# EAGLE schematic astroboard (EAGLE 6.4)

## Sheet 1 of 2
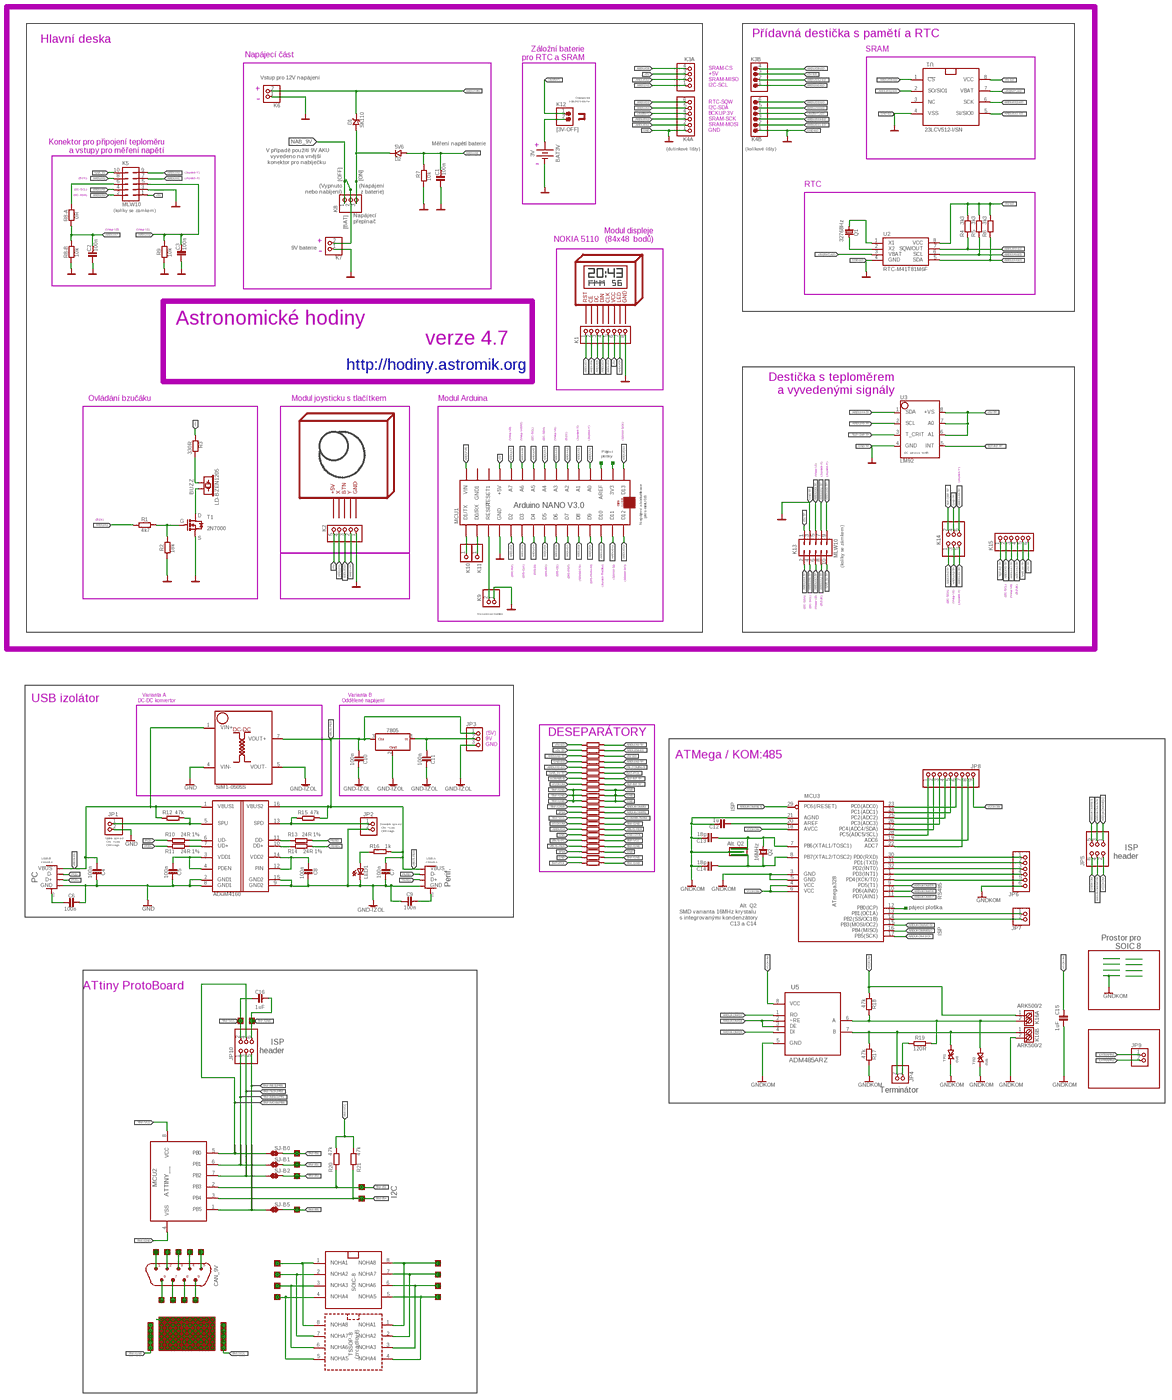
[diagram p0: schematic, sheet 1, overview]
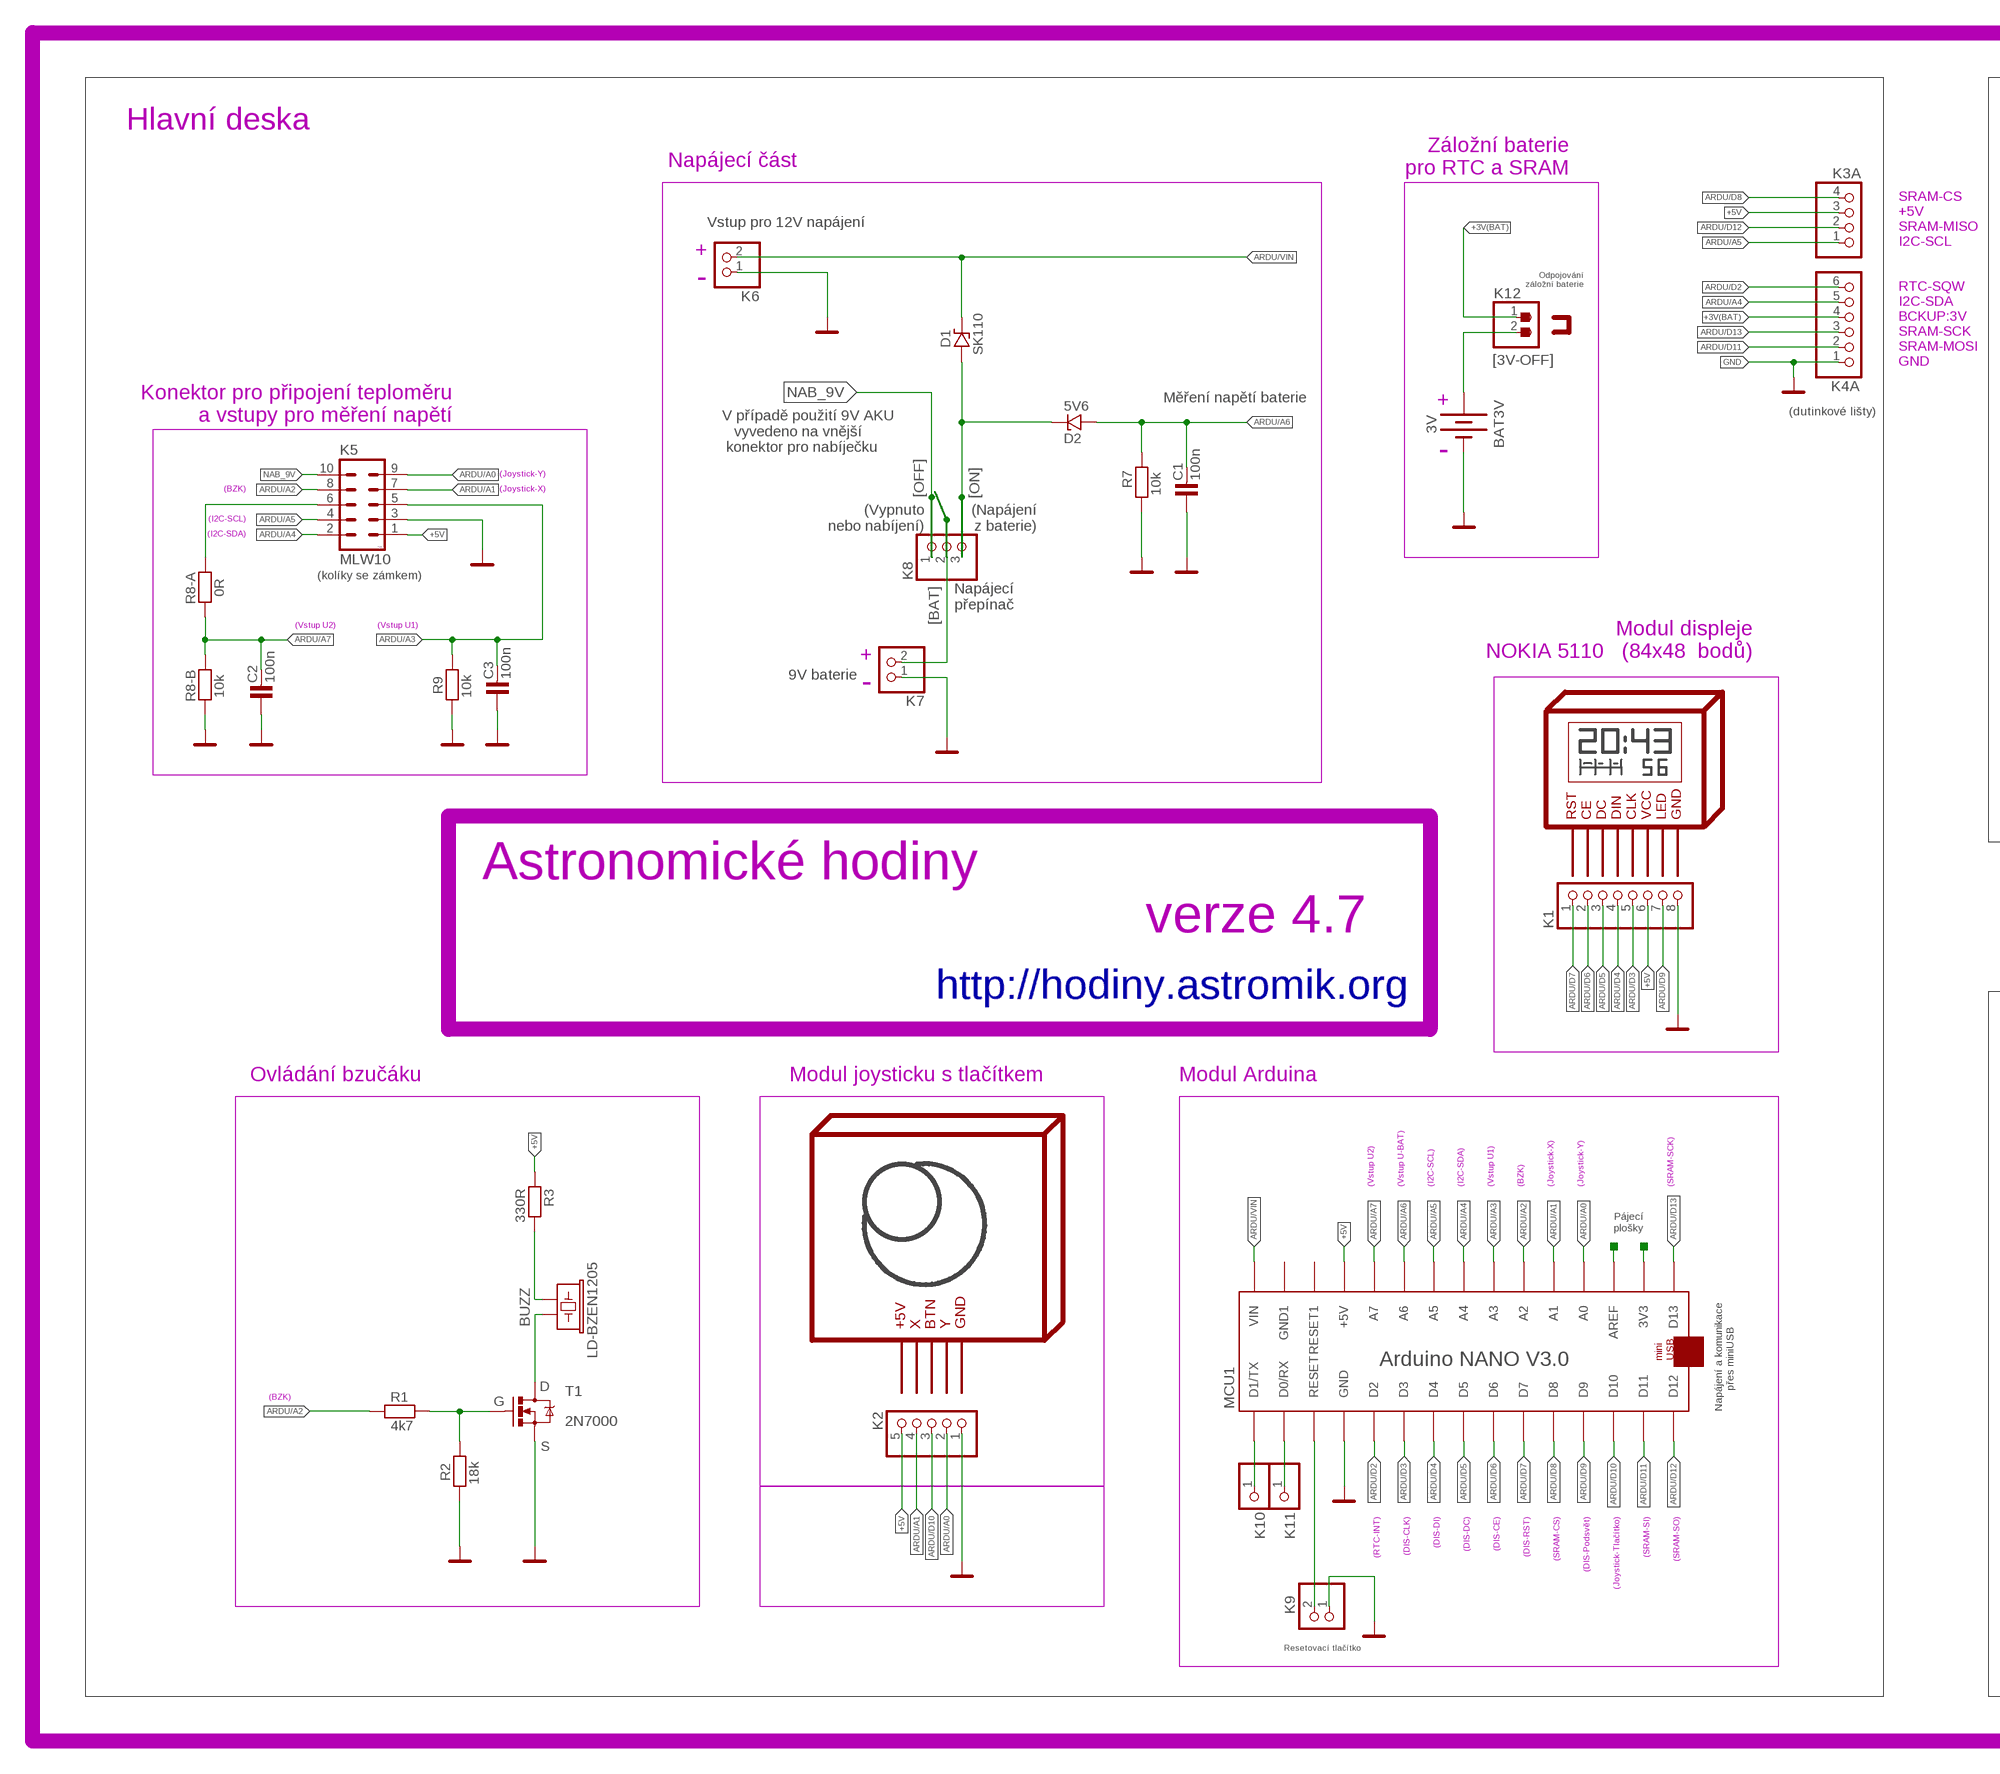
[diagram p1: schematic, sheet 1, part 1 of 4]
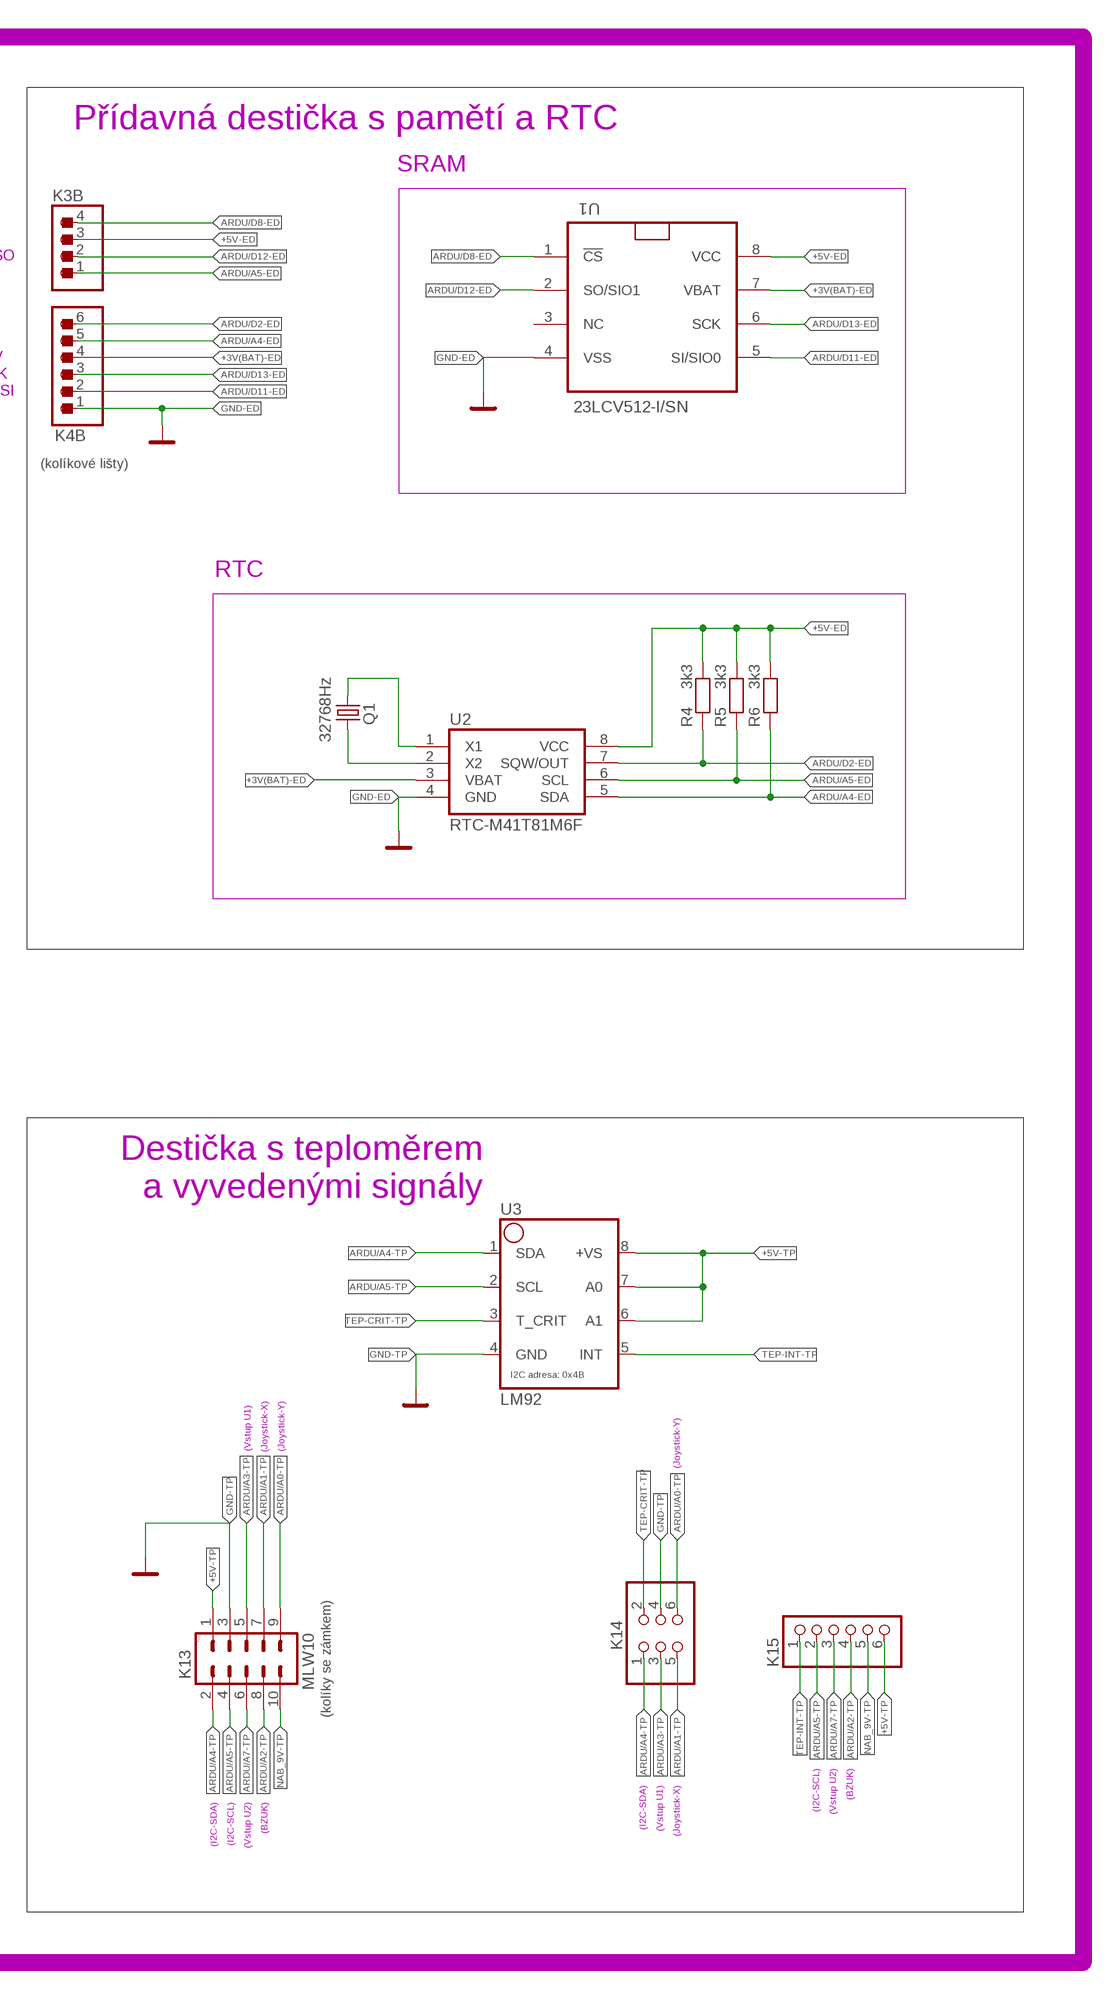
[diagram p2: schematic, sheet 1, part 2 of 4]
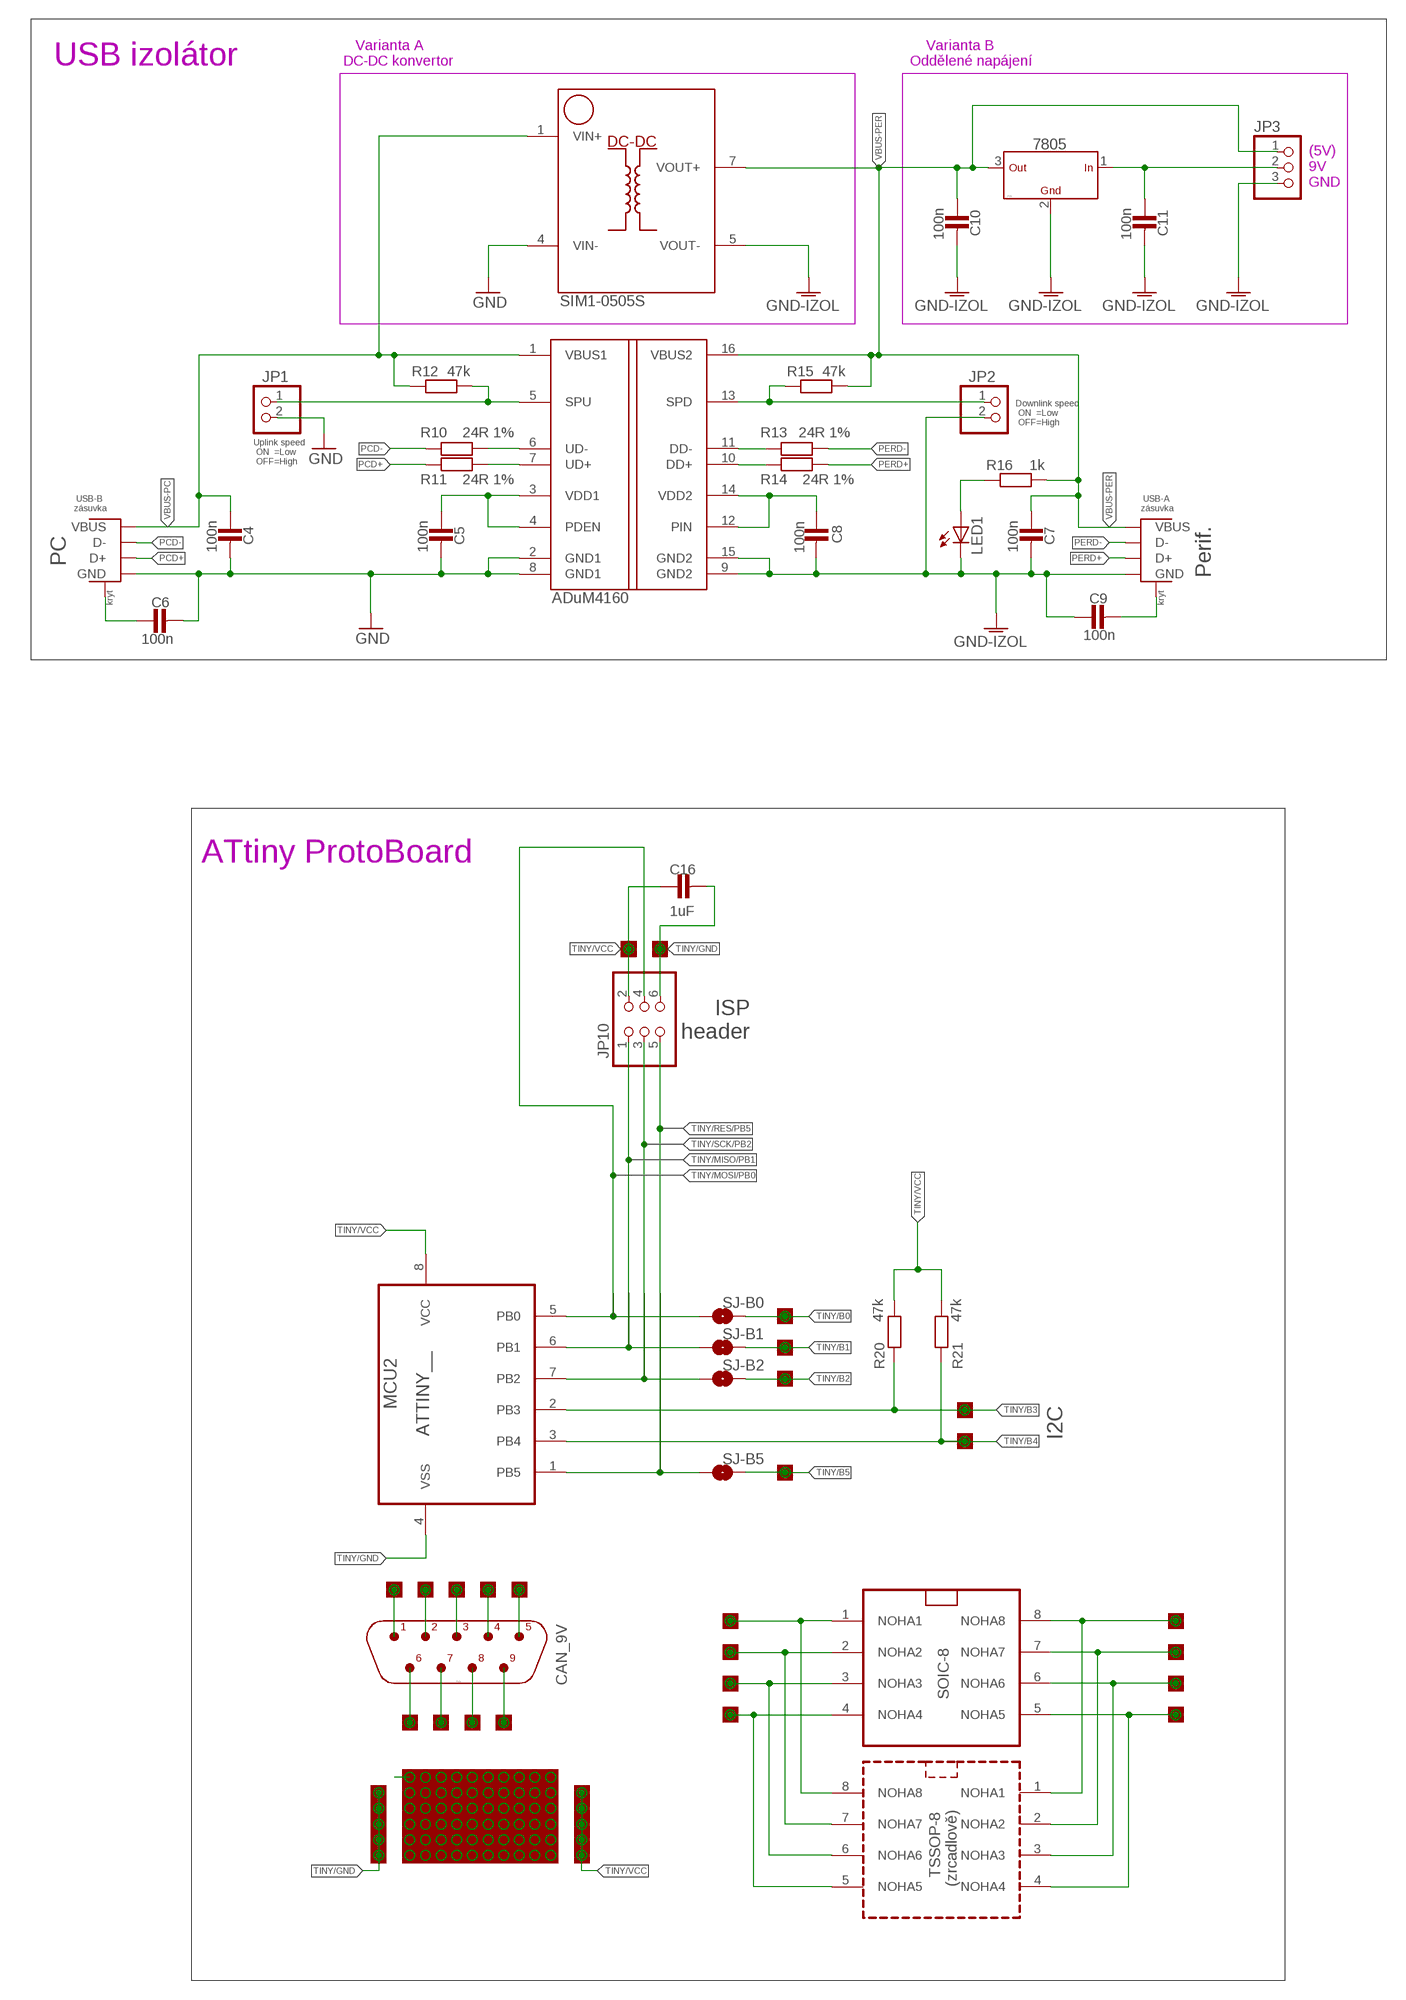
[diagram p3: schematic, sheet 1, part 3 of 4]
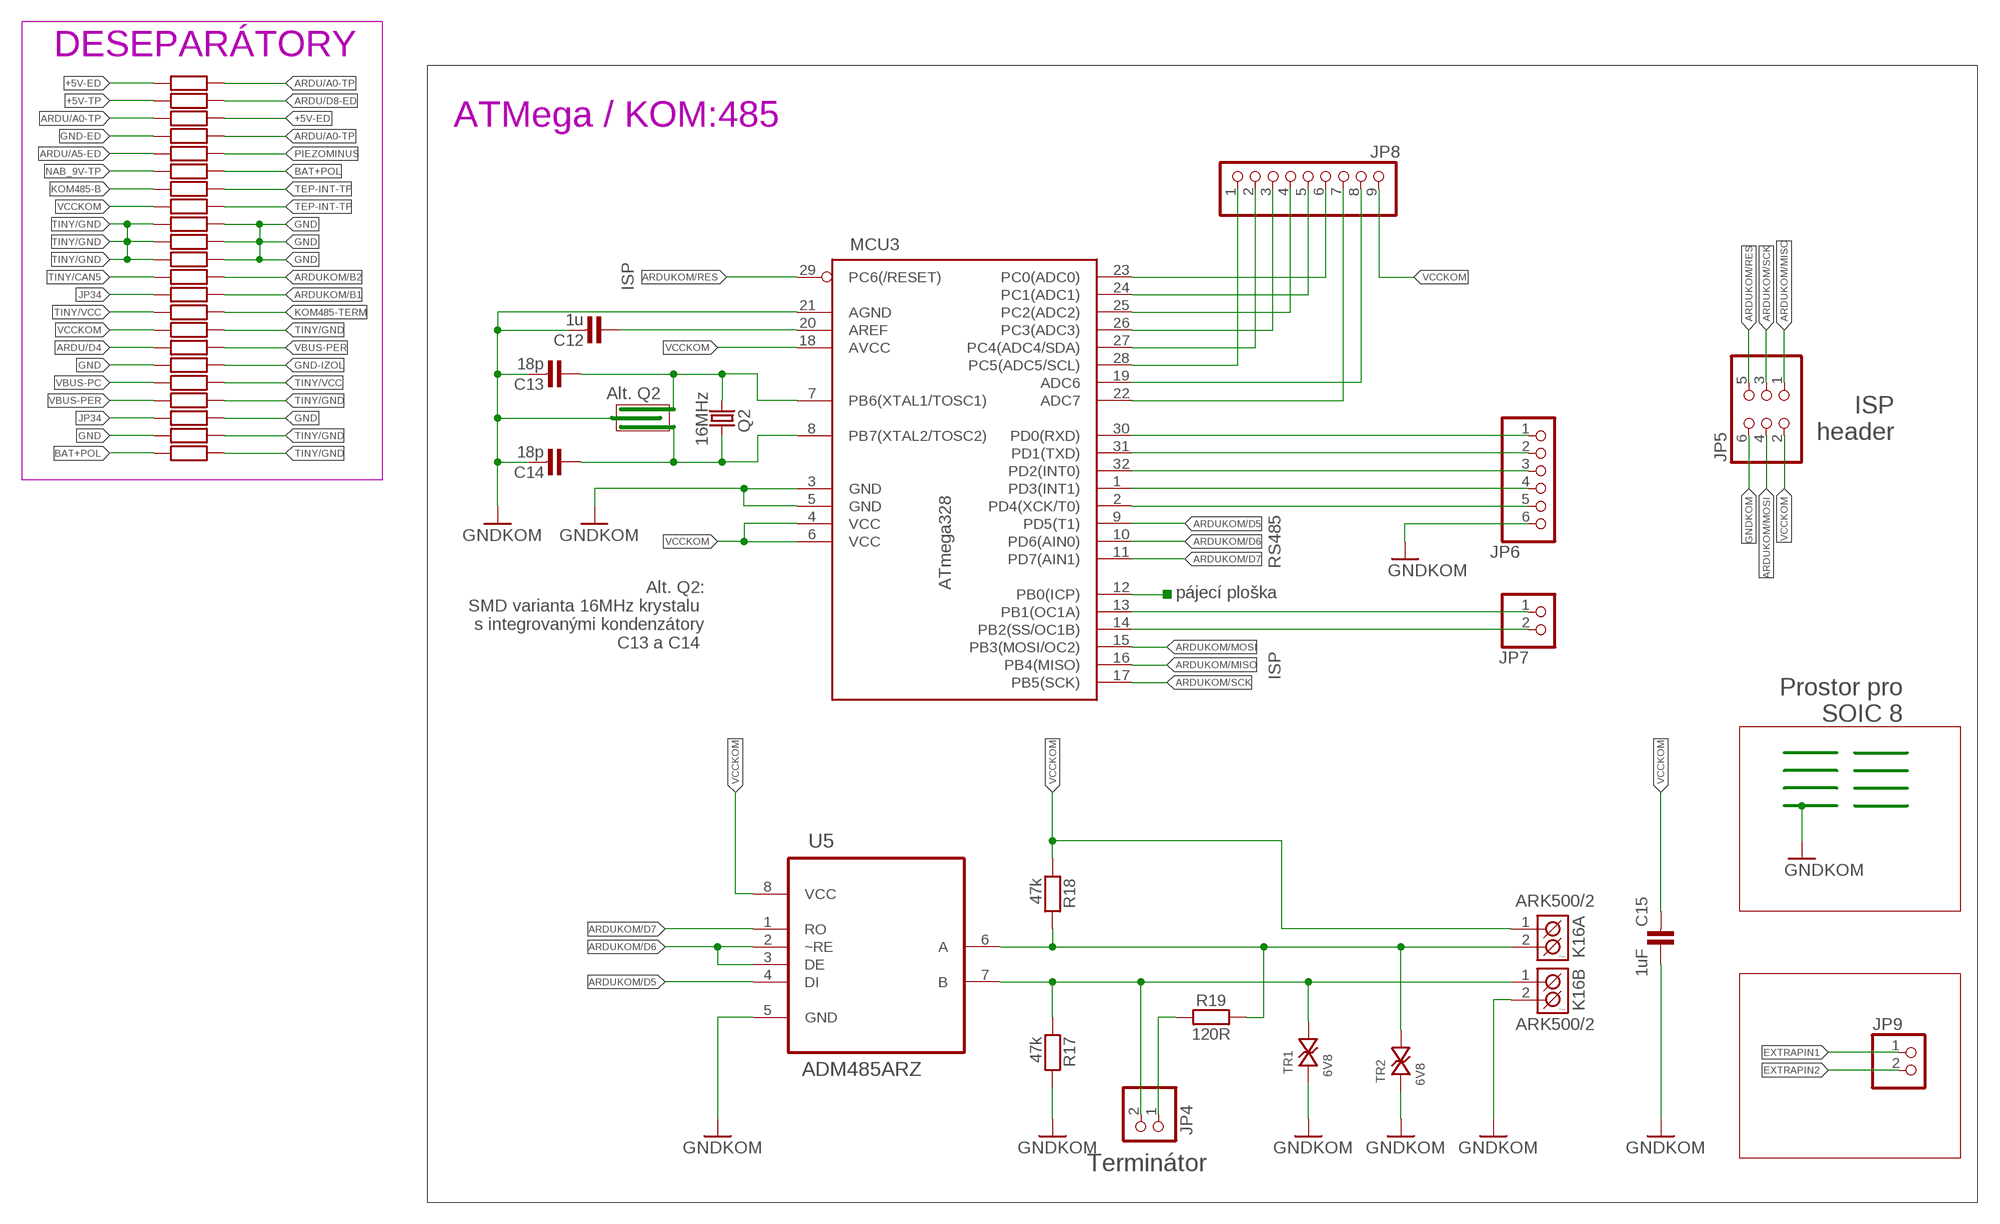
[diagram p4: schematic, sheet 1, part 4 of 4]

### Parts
BAT3V  3V  BATTERY20PTH2  [BATTERY]
BUZZ  LD-BZEN1205  BUZZERNS  [BUZZER-12MM-NS]
C1  100n  C-KERAMIK_SMD_1206  [1206]
C2  100n  C-KERAMIK_SMD_1206  [1206]
C3  100n  C-KERAMIK_SMD_1206  [1206]
C4  100n  C-KERAMIK_SMD_0805  [0805]
C5  100n  C-KERAMIK_SMD_0805  [0805]
C6  100n  C-KERAMIK_SMD_0805  [0805]
C7  100n  C-KERAMIK_SMD_0805  [0805]
C8  100n  C-KERAMIK_SMD_0805  [0805]
C9  100n  C-KERAMIK_SMD_0805  [0805]
C10  100n  C-KERAMIK_SMD_0805  [0805]
C11  100n  C-KERAMIK_SMD_0805  [0805]
C12  1u  C-KERAMIK_SMD_0805  [0805]
C13  18p  C-KERAMIK_SMD_0805  [0805]
C14  18p  C-KERAMIK_SMD_0805  [0805]
C15  1uF  C-KERAMIK_SMD_0805  [0805]
C16  1uF  C-KERAMIK_SMD_0805  [0805]
CAN1  CAN_9V  CAN_9V_/0  [CAN9V]
D1  SK110  1N4007_SM-1  [SM-1]
D2  5V6  D-ZENEROVA_0,5W_BZV55C_SMD  [SOD-80]
DC-DC1  SIM1-0505  [SIM1-0505]
EMPTY1  SOIC-NIC  [SOIC127P600X175-8N]
EMPTY2  TSSOP-NIC  [TSSOP8]
IO1  7805  78_STOJ_STOJ  [TO-220S]
JP1  PINHD-1X2  [1X02]
JP2  PINHD-1X2  [1X02]
JP3  PINHD-1X3  [1X03]
JP4  PINHD-1X2  [1X02]
JP5  PINHD-2X3  [2X03]
JP6  PINHD-1X6  [1X06]
JP7  PINHD-1X2  [1X02]
JP8  PINHD-1X9  [1X09]
JP9  PINHD-1X2  [1X02]
JP10  PINHD-2X3  [2X03]
JP11  PINHD-1X1  [1X01]
JP12  PINHD-1X1  [1X01]
JP13  PINHD-1X1  [1X01]
JP14  PINHD-1X1  [1X01]
JP15  PINHD-1X1  [1X01]
JP16  PINHD-1X1  [1X01]
JP17  PINHD-1X1  [1X01]
JP18  PINHD-1X1  [1X01]
JP19  PINHD-1X1  [1X01]
JP20  PINHD-1X1  [1X01]
JP21  PINHD-1X1  [1X01]
JP22  PINHD-1X1  [1X01]
JP23  PINHD-1X1  [1X01]
JP24  PINHD-1X1  [1X01]
JP25  PINHD-1X1  [1X01]
JP26  PINHD-1X1  [1X01]
JP27  PINHD-1X1  [1X01]
JP28  PINHD-1X1  [1X01]
JP29  PINHD-1X1  [1X01]
JP30  PINHD-1X1  [1X01]
JP31  PINHD-1X1  [1X01]
JP32  PINHD-1X1  [1X01]
JP33  PINHD-1X1  [1X01]
JP34  PINHD-1X1  [1X01]
JP35  PINHD-1X1  [1X01]
JP36  PINHD-1X1  [1X01]
JP37  PINHD-1X1  [1X01]
JP38  PINHD-1X1  [1X01]
JP39  PINHD-1X1  [1X01]
JP40  PINHD-1X1  [1X01]
JP41  PINHD-1X1  [1X01]
JP42  PINHD-1X1  [1X01]
JP43  PINHD-1X1  [1X01]
JP44  PINHD-1X1  [1X01]
JP45  PINHD-1X1  [1X01]
JP46  PINHD-1X1  [1X01]
JP47  PINHD-1X1  [1X01]
JP48  PINHD-1X1  [1X01]
JP49  PINHD-1X1  [1X01]
JP50  PINHD-1X1  [1X01]
JP51  PINHD-1X1  [1X01]
JP52  PINHD-1X1  [1X01]
JP53  PINHD-1X1  [1X01]
JP54  PINHD-1X1  [1X01]
JP55  PINHD-1X1  [1X01]
JP56  PINHD-1X1  [1X01]
JP57  PINHD-1X1  [1X01]
JP58  PINHD-1X1  [1X01]
JP59  PINHD-1X1  [1X01]
JP60  PINHD-1X1  [1X01]
JP61  PINHD-1X1  [1X01]
JP62  PINHD-1X1  [1X01]
JP63  PINHD-1X1  [1X01]
JP64  PINHD-1X1  [1X01]
JP65  PINHD-1X1  [1X01]
JP66  PINHD-1X1  [1X01]
JP67  PINHD-1X1  [1X01]
JP68  PINHD-1X1  [1X01]
JP69  PINHD-1X1  [1X01]
JP70  PINHD-1X1  [1X01]
JP71  PINHD-1X1  [1X01]
JP72  PINHD-1X1  [1X01]
JP73  PINHD-1X1  [1X01]
JP74  PINHD-1X1  [1X01]
JP75  PINHD-1X1  [1X01]
JP76  PINHD-1X1  [1X01]
JP77  PINHD-1X1  [1X01]
JP78  PINHD-1X1  [1X01]
JP79  PINHD-1X1  [1X01]
JP80  PINHD-1X1  [1X01]
JP81  PINHD-1X1  [1X01]
JP82  PINHD-1X1  [1X01]
JP83  PINHD-1X1  [1X01]
JP84  PINHD-1X1  [1X01]
JP85  PINHD-1X1  [1X01]
JP86  PINHD-1X1  [1X01]
JP87  PINHD-1X1  [1X01]
JP88  PINHD-1X1  [1X01]
JP89  PINHD-1X1  [1X01]
JP90  PINHD-1X1  [1X01]
JP91  PINHD-1X1  [1X01]
JP92  PINHD-1X1  [1X01]
JP93  PINHD-1X1  [1X01]
JP94  PINHD-1X1  [1X01]
JP95  PINHD-1X1  [1X01]
JP97  PINHD-1X1  [1X01]
JP98  PINHD-1X1  [1X01]
JP99  PINHD-1X1  [1X01]
JP100  PINHD-1X1  [1X01]
JP101  PINHD-1X1  [1X01]
JP103  PINHD-1X1  [1X01]
JP104  PINHD-1X1  [1X01]
JP105  PINHD-1X1  [1X01]
JP106  PINHD-1X1  [1X01]
JP108  PINHD-1X1  [1X01]
K1  PINHD-1X8  [1X08]
K2  PINHD-1X5  [1X05]
K3A  PINHD-1X4  [1X04]
K3B  PINHD-1X4  [1X04]
K4A  PINHD-1X6  [1X06]
K4B  PINHD-1X6  [1X06]
K5  MLW10  [MLW10G]
K6  PINHD-1X2  [1X02]
K7  HEADER-1X2  [1X02_OVAL]
K8  PINHD-1X3  [1X03]
K9  PINHD-1X2  [1X02]
K10  PINHD-1X1  [1X01]
K11  PINHD-1X1  [1X01]
K12  PINHD-1X2  [1X02]
K13  MLW10  [MLW10G]
K14  PINHD-2X3  [2X03]
K15  PINHD-1X6  [1X06]
K16A  ARK500/2  [ARK500/2]
K16B  ARK500/2  [ARK500/2]
LED1  LEDCHIP-LED0805  [CHIP-LED0805]
MCU1  ARDUINONANO  [PDIP-32]
MCU2  ATTINY__  ATTINY13  [SOIC127P600X175-8N]
MCU3  ATmega328  MEGA8-AI  [TQFP32-08]
Q1  32768Hz  CRYSTALTC26V  [TC26V]
Q2  16MHz  CRYSTALHC49U-V  [HC49U-V]
R1  4k7  R_SMD_1206  [1206]
R2  18k  R_SMD_1206  [1206]
R3  330R  R_SMD_1206  [1206]
R4  3k3  R_SMD_1206  [1206]
R5  3k3  R_SMD_1206  [1206]
R6  3k3  R_SMD_1206  [1206]
R7  10k  R_SMD_1206  [1206]
R8  1k  R_SMD_1206  [1206]
R8-A  0R  R_SMD_1206  [1206]
R8-B  10k  R_SMD_1206  [1206]
R9  10k  R_SMD_1206  [1206]
R10  24R 1%  R_SMD_0805  [0805]
R11  24R 1%  R_SMD_0805  [0805]
R12  47k  R_SMD_0805  [0805]
R13  24R 1%  R_SMD_0805  [0805]
R14  24R 1%  R_SMD_0805  [0805]
R15  47k  R_SMD_0805  [0805]
R16  1k  R_SMD_0805  [0805]
R17  47k  R_SMD_0805  [0805]
R18  47k  R_SMD_0805  [0805]
R19  120R  R_SMD_0805  [0805]
R20  47k  R_SMD_0805  [0805]
R21  47k  R_SMD_0805  [0805]
R22  1k  R_SMD_1206  [1206]
R23  1k  R_SMD_1206  [1206]
R24  1k  R_SMD_1206  [1206]
R25  1k  R_SMD_1206  [1206]
R26  1k  R_SMD_1206  [1206]
R27  1k  R_SMD_1206  [1206]
R28  1k  R_SMD_1206  [1206]
R29  1k  R_SMD_1206  [1206]
R30  1k  R_SMD_1206  [1206]
R31  1k  R_SMD_1206  [1206]
R32  1k  R_SMD_1206  [1206]
R33  1k  R_SMD_1206  [1206]
R34  1k  R_SMD_1206  [1206]
R35  1k  R_SMD_1206  [1206]
R36  1k  R_SMD_1206  [1206]
R37  1k  R_SMD_1206  [1206]
R38  1k  R_SMD_1206  [1206]
R39  1k  R_SMD_1206  [1206]
R40  1k  R_SMD_1206  [1206]
R41  1k  R_SMD_1206  [1206]
R42  1k  R_SMD_1206  [1206]
SJ-B0  SOLDERJUMPERNC  [SJ-NC]
SJ-B1  SOLDERJUMPERNC  [SJ-NC]
SJ-B2  SOLDERJUMPERNC  [SJ-NC]
SJ-B5  SOLDERJUMPERNC  [SJ-NC]
T1  2N7000  MOSFET-NCHANNELPTH  [TO-92]
TR1  6V8  SMAJ30CA-TR__DO214AC+MINIMELF  [DO214AC+MINIMELF_BIDIR]
TR2  6V8  SMAJ30CA-TR__DO214AC+MINIMELF  [DO214AC+MINIMELF_BIDIR]
U1  23LCV512-I/SN  [SOIC127P600X175-8N]
U2  RTC-M41T81M6F  IC_RTC_DS1307  [SO-8]
U3  LM92  [SO08]
U4  ADuM4160  ADUM4160  [SO16W]
U5  ADM485ARZ  [SOIC127P600X175-8N]
X1  USB B  USBPTH  [USB-B-PTH]
X2  USB A  USBA-H  [USB-A-H]

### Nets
+3V(BAT): K4A.4 K12.1
+3V(BAT)-ED: K4B.4 U1.7(VBAT) U2.3(VBAT)
+5V: K1.6 K2.5 K3A.3 K5.1 MCU1.+5V R3.1
+5V-ED: K3B.3 R4.2 R5.2 R6.2 R8.1 R33.2 U1.8(VCC) U2.8(VCC)
+5V-TP: K13.1 K15.6 R25.2 U3.6(A1) U3.7(A0) U3.8(+VS)
ARDU/3V3: MCU1.3V3
ARDU/A0: K2.2 K5.9 MCU1.A0
ARDU/A0-TP: K13.9 K14.6 R8.2 R22.1 R33.1
ARDU/A1: K2.4 K5.7 MCU1.A1
ARDU/A1-TP: K13.7 K14.5
ARDU/A2: K5.8 MCU1.A2 R1.1
ARDU/A2-TP: K13.8 K15.4
ARDU/A3: C3.2 K5.5 MCU1.A3 R9.2
ARDU/A3-TP: K13.5 K14.3
ARDU/A4: K4A.5 K5.2 MCU1.A4
ARDU/A4-ED: K4B.5 R6.1 U2.5(SDA)
ARDU/A4-TP: K13.2 K14.1 U3.1(SDA)
ARDU/A5: K3A.1 K5.4 MCU1.A5
ARDU/A5-ED: K3B.1 R5.1 R23.2 U2.6(SCL)
ARDU/A5-TP: K13.4 K15.2 U3.2(SCL)
ARDU/A6: C1.2 D2.A MCU1.A6 R7.2
ARDU/A7: C2.2 MCU1.A7 R8-A.1 R8-B.2
ARDU/A7-TP: K13.6 K15.3
ARDU/AREF: MCU1.AREF
ARDU/D0: K11.1 MCU1.D0/RX
ARDU/D1: K10.1 MCU1.D1/TX
ARDU/D2: K4A.6 MCU1.D2
ARDU/D2-ED: K4B.6 R4.1 U2.7(SQW/OUT)
ARDU/D3: K1.5 MCU1.D3
ARDU/D4: K1.4 MCU1.D4 R36.2
ARDU/D5: K1.3 MCU1.D5
ARDU/D6: K1.2 MCU1.D6
ARDU/D7: K1.1 MCU1.D7
ARDU/D8: K3A.4 MCU1.D8
ARDU/D8-ED: K3B.4 R25.1 U1.1(!CS)
ARDU/D9: K1.7 MCU1.D9
ARDU/D10: K2.3 MCU1.D10
ARDU/D11: K4A.2 MCU1.D11
ARDU/D11-ED: K4B.2 U1.5(SI/SIO0)
ARDU/D12: K3A.2 MCU1.D12
ARDU/D12-ED: K3B.2 U1.2(SO/SIO1)
ARDU/D13: K4A.3 MCU1.D13
ARDU/D13-ED: K4B.3 U1.6(SCK)
ARDU/RESET: K9.2 MCU1.RESET
ARDU/VIN: D1.K K6.2 MCU1.VIN
ARDUKOM/B0: MCU3.12(PB0(ICP))
ARDUKOM/B1: JP7.1 MCU3.13(PB1(OC1A)) R32.1
ARDUKOM/B2: JP7.2 MCU3.14(PB2(SS/OC1B)) R30.1
ARDUKOM/C0: JP8.6 MCU3.23(PC0(ADC0))
ARDUKOM/C1: JP8.5 MCU3.24(PC1(ADC1))
ARDUKOM/C2: JP8.4 MCU3.25(PC2(ADC2))
ARDUKOM/C3: JP8.3 MCU3.26(PC3(ADC3))
ARDUKOM/C4: JP8.2 MCU3.27(PC4(ADC4/SDA))
ARDUKOM/C5: JP8.1 MCU3.28(PC5(ADC5/SCL))
ARDUKOM/C6: JP8.8 MCU3.19(ADC6)
ARDUKOM/C7: JP8.7 MCU3.22(ADC7)
ARDUKOM/D0: JP6.1 MCU3.30(PD0(RXD))
ARDUKOM/D1: JP6.2 MCU3.31(PD1(TXD))
ARDUKOM/D2: JP6.3 MCU3.32(PD2(INT0))
ARDUKOM/D3: JP6.4 MCU3.1(PD3(INT1))
ARDUKOM/D4: JP6.5 MCU3.2(PD4(XCK/T0))
ARDUKOM/D5: MCU3.9(PD5(T1)) U5.4(DI)
ARDUKOM/D6: MCU3.10(PD6(AIN0)) U5.2(~RE) U5.3(DE)
ARDUKOM/D7: MCU3.11(PD7(AIN1)) U5.1(RO)
ARDUKOM/MISO: JP5.1 MCU3.16(PB4(MISO))
ARDUKOM/MOSI: JP5.4 MCU3.15(PB3(MOSI/OC2))
ARDUKOM/RES: JP5.5 MCU3.29(PC6(/RESET))
ARDUKOM/SCK: JP5.3 MCU3.17(PB5(SCK))
BAT+POL: BAT3V.+ K12.2 R24.1 R42.2
BZUK/GATE: R1.2 R2.2 T1.3(G)
EXTRAPIN1: JP9.1
EXTRAPIN2: JP9.2
GND: BAT3V.- C1.1 C2.1 C3.1 K1.8 K2.1 K4A.1 K5.3 K6.1 K7.1 K9.1 MCU1.GND R2.1 R7.1 R8-B.1 R9.1 R27.1 R28.1 R29.1 R37.2 R40.1 R41.2 T1.1(S)
GND-ED: K4B.1 R22.2 U1.4(VSS) U2.4(GND) ; supply symbol labelled GND
GND-IZOL: C7.2 C8.2 C9.1 C10.2 C11.2 DC-DC1.5(VOUT-) IO1.2(GND) JP2.2 JP3.3 LED1.C R37.1 U4.9(GND2) U4.15(GND2) X2.GND
GND-PC: C4.2 C5.2 C6.2 DC-DC1.4(VIN-) JP1.2 U4.2(GND1) U4.8(GND1) X1.GND ; supply symbol labelled GND
GND-TP: K13.3 K14.4 U3.4(GND) ; supply symbol labelled GND
GNDKOM: C12.2 C13.2 C14.2 C15.1 JP5.6 JP6.6 K16B.2(K2) MCU3.3(GND) MCU3.5(GND) MCU3.21(AGND) R17.2 TR1.P$1 TR2.P$1 U5.5(GND)
JP34: JP34.1 R32.2 R40.2
KOM485-A: K16A.2(K2) R18.2 R19.2 TR2.P$2 U5.6(A)
KOM485-B: JP4.2 K16B.1(K1) R17.1 R26.2 TR1.P$2 U5.7(B)
KOM485-TERM: JP4.1 R19.1 R34.1
N$1: K5.6 R8-A.2
N$2: C6.1 X1.P$2(SHIELD)
N$3: R11.2 U4.7(UD+)
N$4: R10.2 U4.6(UD-)
N$5: C9.2 X2.SHIELD@1(SHIELD)
N$9: JP1.1 R12.1 U4.5(SPU)
N$10: JP2.1 R15.1 U4.13(SPD)
N$14: R14.1 U4.10(DD+)
N$15: C11.1 IO1.1(IN) JP3.2
N$16: R13.1 U4.11(DD-)
N$18: LED1.A R16.1
N$21: C13.1 MCU3.7(PB6(XTAL1/TOSC1)) Q2.2
N$22: C14.1 MCU3.8(PB7(XTAL2/TOSC2)) Q2.1
N$28: C12.1 MCU3.20(AREF)
NAB_9V: K5.10 K8.1
NAB_9V-TP: K13.10 K15.5 R24.2
NAPETI_9V: D1.A D2.K K8.3
OSC1-ED: Q1.2 U2.1(X1)
OSC2-ED: Q1.1 U2.2(X2)
PCD+: R11.1 X1.D+
PCD-: R10.1 X1.D-
PERD+: R14.2 X2.D+
PERD-: R13.2 X2.D-
PIEZOMINUS: BUZZ.- R23.1 T1.2(D)
PIEZOPLUS: BUZZ.+ R3.2
PLUS_9V: K7.2 K8.2
TEP-CRIT-TP: K14.2 U3.3(T_CRIT)
TEP-INT-TP: K15.1 R26.1 R31.1 U3.5(INT)
TINY/B0: JP27.1 SJ-B0.2
TINY/B1: JP28.1 SJ-B1.2
TINY/B2: JP29.1 SJ-B2.2
TINY/B3: JP31.1 MCU2.2(PB3) R20.1
TINY/B4: JP32.1 MCU2.3(PB4) R21.1
TINY/B5: JP30.1 SJ-B5.2
TINY/CAN1: CAN1.1 JP18.1
TINY/CAN2: CAN1.2 JP19.1
TINY/CAN3: CAN1.3 JP20.1
TINY/CAN4: CAN1.4 JP21.1
TINY/CAN5: CAN1.5 JP22.1 R30.2
TINY/CAN6: CAN1.6 JP23.1
TINY/CAN7: CAN1.7 JP24.1
TINY/CAN8: CAN1.8 JP25.1
TINY/CAN9: CAN1.9 JP26.1
TINY/GND: C16.2 JP10.6 JP93.1 JP94.1 JP97.1 JP98.1 JP99.1 JP100.1 MCU2.4(VSS) R27.2 R28.2 R29.2 R35.1 R39.1 R41.1 R42.1
TINY/MISO/PB1: JP10.1 MCU2.6(PB1) SJ-B1.1
TINY/MOSI/PB0: JP10.4 MCU2.5(PB0) SJ-B0.1
TINY/RES/PB5: JP10.5 MCU2.1(PB5) SJ-B5.1
TINY/SCK/PB2: JP10.3 MCU2.7(PB2) SJ-B2.1
TINY/SOIC1: EMPTY1.1(NOHA1) EMPTY2.8(NOHA8) JP14.1
TINY/SOIC2: EMPTY1.2(NOHA2) EMPTY2.7(NOHA7) JP15.1
TINY/SOIC3: EMPTY1.3(NOHA3) EMPTY2.6(NOHA6) JP16.1
TINY/SOIC4: EMPTY1.4(NOHA4) EMPTY2.5(NOHA5) JP17.1
TINY/SOIC5: EMPTY1.5(NOHA5) EMPTY2.4(NOHA4) JP13.1
TINY/SOIC6: EMPTY1.6(NOHA6) EMPTY2.3(NOHA3) JP12.1
TINY/SOIC7: EMPTY1.7(NOHA7) EMPTY2.2(NOHA2) JP11.1
TINY/SOIC8: EMPTY1.8(NOHA8) EMPTY2.1(NOHA1) JP108.1
TINY/VCC: C16.1 JP10.2 JP95.1 JP101.1 JP103.1 JP104.1 JP105.1 JP106.1 MCU2.8(VCC) R20.2 R21.2 R34.2 R38.1
VBUS-PC: C4.1 DC-DC1.1(VIN+) R12.2 R38.2 U4.1(VBUS1) X1.VBUS
VBUS-PER: C7.1 C10.1 DC-DC1.7(VOUT+) IO1.3(OUT) JP3.1 R15.2 R16.2 R36.1 R39.2 U4.16(VBUS2) X2.VBUS
VCCKOM: C15.2 JP5.2 JP8.9 K16A.1(K1) MCU3.4(VCC) MCU3.6(VCC) MCU3.18(AVCC) R18.1 R31.2 R35.2 U5.8(VCC)
VDD1: C5.1 U4.3(VDD1) U4.4(PDEN)
VDD2: C8.1 U4.12(PIN) U4.14(VDD2)
Unconnected: JP33.1 JP35.1 JP36.1 JP37.1 JP38.1 JP39.1 JP40.1 JP41.1 JP42.1 JP43.1 JP44.1 JP45.1 JP46.1 JP47.1 JP48.1 JP49.1 JP50.1 JP51.1 JP52.1 JP53.1 JP54.1 JP55.1 JP56.1 JP57.1 JP58.1 JP59.1 JP60.1 JP61.1 JP62.1 JP63.1 JP64.1 JP65.1 JP66.1 JP67.1 JP68.1 JP69.1 JP70.1 JP71.1 JP72.1 JP73.1 JP74.1 JP75.1 JP76.1 JP77.1 JP78.1 JP79.1 JP80.1 JP81.1 JP82.1 JP83.1 JP84.1 JP85.1 JP86.1 JP87.1 JP88.1 JP89.1 JP90.1 JP91.1 JP92.1 MCU1.GND1 MCU1.RESET1 U1.3(NC)

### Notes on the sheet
- Přídavná destička s pamětí a RTC
- Hlavní deska
- Záložní baterie
   pro RTC a SRAM
- SRAM
- Napájecí část
- SRAM-CS
- +5V
- Vstup pro 12V napájení | SRAM-MISO
- + | I2C-SCL
- -
- Odpojování
   záložní baterie
- RTC-SQW
- I2C-SDA
- BCKUP:3V
- SRAM-SCK
- [3V-OFF] | SRAM-MOSI
- GND
- Konektor pro připojení teploměru
  a vstupy pro měření napětí
- Měření napětí baterie | +
- (dutinkové lišty) | (kolíkové lišty)
- -
- V případě použití 9V AKU
     vyvedeno na vnější
   konektor pro nabíječku
- [ON]
- (Joystick-Y)
- (BZK) | (Joystick-X)
- [OFF] | RTC
- (Vypnuto
   nebo nabíjení)
- (Napájení
  z baterie)
- (I2C-SCL)
- (I2C-SDA)
- (kolíky se zámkem)
- Napájecí
  přepínač
- Modul displeje
  NOKIA 5110   (84x48  bodů)
- [BAT]
- (Vstup U2) | (Vstup U1)
- +
- 9V baterie | -
- RST | CE | DC | DIN | CLK | VCC | LED | GND
- Astronomické hodiny | verze 4.7
- http://hodiny.astromik.org
- Destička s teploměrem
  a vyvedenými signály
- Ovládání bzučáku | Modul joysticku s tlačítkem | Modul Arduina
- (Vstup U2) | (Vstup U-BAT) | (I2C-SCL) | (I2C-SDA) | (Vstup U1) | (BZK) | (Joystick-X) | (Joystick-Y) | (SRAM-SCK)
- I2C adresa: 0x4B
- Pájecí
  plošky
- (Joystick-X) | (Joystick-Y)
- (Vstup U1)
- (Joystick-Y)
- +5V | X | BTN | Y | GND
- Arduino NANO V3.0
- MCU1
- D
- G
- (BZK)
- Napájení a komunikace
         přes miniUSB
- S
- (RTC-INT) | (DIS-CLK) | (DIS-DI) | (DIS-DC) | (DIS-CE) | (DIS-RST) | (SRAM-CS) | (DIS-Podsvět) | (Joystick-Tlačítko) | (SRAM-SI) | (SRAM-SO)
- (kolíky se zámkem)
- (I2C-SCL) | (Vstup U2) | (BZUK)
- (I2C-SDA) | (Vstup U1) | (Joystick-X)
- (I2C-SDA) | (I2C-SCL) | (Vstup U2) | (BZUK)
- Resetovací tlačítko
- USB izolátor
- Varianta A
  DC-DC konvertor
- Varianta B
  Oddělené napájení
- DESEPARÁTORY
- (5V)
- 9V
- GND
- ATMega / KOM:485
- ISP
- Downlink speed
   ON  =Low
   OFF=High
- Alt. Q2
- ISP
  header
- Uplink speed
   ON  =Low
   OFF=High
- USB-B
  zásuvka
- USB-A
  zásuvka
- PC | RS485
- Perif.
- kryt | kryt
- Alt. Q2:
    SMD varianta 16MHz krystalu 
    s integrovanými kondenzátory
    C13 a C14
- pájecí ploška
- ISP
- Prostor pro
     SOIC 8
- ATtiny ProtoBoard
- ISP
  header
- Terminátor
- I2C
- SOIC-8
- TSSOP-8
  (zrcadlově)

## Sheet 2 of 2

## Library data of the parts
BAT3V = SparkFun:BATTERY: Battery Holders
BUZZ = SparkFun:BUZZER: Buzzer 12mm
C1-C16 = #PaJa_30:C-KERAMIK: Kondenzator - keramicky
CAN1 = #PaJa_konektory:CAN_9V: Konektory CANNON - vidlice - 9pinu
D1 = #PaJa_30:1N4007: Usmernovaci dioda - 1A, 1000V
D2 = #PaJa_30:D-ZENEROVA: Zenerova dioda
DC-DC1 = sim1-0505:SIM1-0505: DC-DC converter 5V/200mA
EMPTY1 = soic-nic:SOIC-NIC: SOIC-NIC; PACKAGE: SOIC-8
EMPTY2 = tssop-nic:TSSOP-NIC: TSSOP-NIC; PACKAGE: TSSOP-8
IO1 = #PaJa_30:78??: Stabilizátor - 1A a 1,5A ?? - napeti => 05, 06, 08, 09, 12, 15, 18, 20, 24 => 1,5A ?? - napeti => 10, 12, 15, 18 => 1A S ?? - napeti => 05, 09, 10, 12, 15, 18, 24 => 2A T ?? - napeti => 05 => 3A
JP1 JP2 JP4 JP7 JP9 K6 K9 = pinhead:PINHD-1X2: PIN HEADER
JP3 K8 = pinhead:PINHD-1X3: PIN HEADER
JP5 JP10 K14 = pinhead:PINHD-2X3: PIN HEADER
JP6 K4A K15 = pinhead:PINHD-1X6: PIN HEADER
JP8 = pinhead:PINHD-1X9: PIN HEADER
JP11-JP95 JP97-JP101 JP103-JP106 JP108 = jedenpin:PINHD-1X1: PIN HEADER
K1 = pinhead:PINHD-1X8: PIN HEADER
K2 = pinhead:PINHD-1X5: PIN HEADER
K3A = pinhead:PINHD-1X4: PIN HEADER
K3B = pinhead-rev:PINHD-1X4: PIN HEADER
K4B = pinhead-rev:PINHD-1X6: PIN HEADER
K5 K13 = #PaJa_konektory:MLW10: Konektory MLW - vidlice - 10x
K7 = nonolith:HEADER-1X2: PIN HEADER
K10 K11 = pinhead:PINHD-1X1: PIN HEADER
K12 = pinhead-rev:PINHD-1X2: PIN HEADER
K16A K16B = #PaJa_konektory:ARK500/2: Svorkovnice - roztec 5mm - dvojita
LED1 = adafruit:LED: LED
MCU1 = jet-lib:ARDUINONANO
MCU2 = ATTiny13:ATTINY13: ATTINY13; PACKAGE: SOIC-8
MCU3 = avr:MEGA8: MICROCONTROLLER 8 Kbytes FLASH 1 kbytes SRAM 512 bytes EEPROM USART 6-channel 10 bit ADC 2-channel 8 bit ADC
Q1 = adafruit:CRYSTAL: CRYSTAL; OC_FARNELL: unknown; OC_NEWARK: unknown
Q2 = adafruit:CRYSTAL: CRYSTAL; OC_FARNELL: 1666969; OC_NEWARK: unknown
R1-R8 R8-A R8-B R9-R42 = #PaJa_30:R: Rezistor
SJ-B0 SJ-B1 SJ-B2 SJ-B5 = SparkFun:SOLDERJUMPER: Solder Jumper
T1 = SparkFun:MOSFET-NCHANNEL
TR1 TR2 = transil:SMAJ30CA-TR__DO214AC+MINIMELF: Transil SMAJ 30 Volt BIDIR.
U1 = 23LCV512:23LCV512-I/SN: 512 Kbit SPI Serial SRAM,SOIC-8; MPN: 23LCV512-I/SN; OC_FARNELL: 2309512; OC_NEWARK: 70W1662; PACKAGE: SOIC-8; SUPPLIER: MICROCHIP
U2 = dp_devices:IC_RTC_DS1307
U3 = emile:LM92
U4 = CH_Analog_Devices:ADUM4160: Analog Devices Low/Full Speed USB Isolator
U5 = Analog Devices_By_element14_Batch_1:ADM485ARZ: 5 V Low Power EIA RS-485 Transceiver; MPN: ADM485ARZ; OC_FARNELL: 1661065; OC_NEWARK: 19M8696; PACKAGE: SOIC-8; SUPPLIER: Analog Devices
X1 X2 = CH_connectors:USB: USB Connectors USB-B-PTH is fully proven SKU : PRT-00139 USB-miniB is fully proven SKU : PRT-00587 USB-A-PCB is untested. USB-A-H is C@H proven USB-B-SMT is throughly reviewed, but untested. Needs silkscreen touching up. USB-A-S has not been used/tested USB-MB-H has not been used/tested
